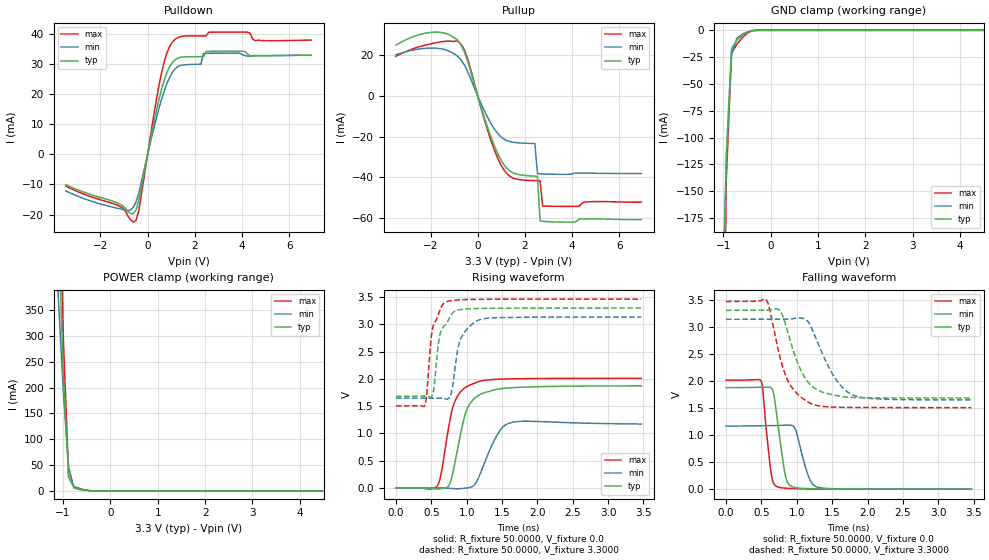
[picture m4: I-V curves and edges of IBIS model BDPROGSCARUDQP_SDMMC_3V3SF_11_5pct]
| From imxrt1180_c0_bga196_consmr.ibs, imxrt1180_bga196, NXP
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[Model]  BDPROGSCARUDQP_SDMMC_3V3SF_11_5pct
|   Model BDPROGSCARUDQP_SDMMC_3V3SF_11_5pct
| This model was characterised for following simulation conditions:
| External (pad) voltage:
|   - Typ: 3.3V,   - Min: 3.135V,   - Max: 3.465V
| Library cells for typ/min/max conditions are connected as defined below:
|  IO - External Pad
|  A - Core Input
|  EN - Output Buffer Enable
|  ASRCN3V3[0] - REFH3V3
|  ASRCN3V3[1] - REFH3V3 REFH3V3 gnde
|  ASRCN3V3[2] - gnde
|  ASRCN3V3[3] - gnde REFH3V3 gnde
|  ASRCP3V3[0] - vdde3v3 REFL3V3 REFL3V3
|  ASRCP3V3[1] - vdde3v3 REFL3V3 vdde3v3
|  ASRCP3V3[2] - REFL3V3 vdde3v3 vdde3v3
|  ASRCP3V3[3] - REFL3V3 REFL3V3 vdde3v3
|  IOGC - NC
|  PDN - vdd
|  PDRV - vdd
|  PSW - vdd
|  PUN - vdd
|  REFH3V3 - REFH3V3
|  REFL3V3 - REFL3V3
|  ZI - NC
|  gnd - gnd
|  gnde - gnde
|  vdd - vdd
|  vdde3v3 - vdde3v3
| All other pins connected to ground
Model_type I/O
Polarity   Non-Inverting
Enable   Active-Low
Vinl =   0.7500V
Vinh =   2.2500V
Vmeas =  1.6500V
Cref =   30.0000pF
Rref =   1.0000M
Vref =   3.3000V
C_comp   2.0930pF   2.0578pF   2.1401pF
|C_comp_pullup   0.3785pF   0.3910pF   0.3686pF
|C_comp_pulldown   0.6262pF   0.6569pF   0.6008pF
[Model Spec]
| variable   typ   min   max
Vinh   2.0625V   1.9594V   2.1656V
Vinl   0.8250V   0.7837V   0.8662V
[Temperature Range]   25.0000   0.1050k   -20.0000
[Voltage Range]   3.3000V   3.1350V   3.4650V
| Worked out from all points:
|   slope of the pulldown table from 0 to 0.495 V, typ, clamps not added: 26.6 ohm
|   slope of the pullup table from 0 to 0.495 V, typ, clamps not added: 27.4 ohm
|   GND clamp passes 1 mA (typ) near -0.44 V on its own axis
|   POWER clamp passes 1 mA (typ) near -0.50 V on its own axis
|   rising waveform, R_fixture 50.0000, V_fixture 0.0: 20-80 % time 205ps typ, 233ps min, 182ps max; typ from 0 V to 1.87 V
|   rising waveform, R_fixture 50.0000, V_fixture 3.3000: 20-80 % time 135ps typ, 150ps min, 118ps max; typ from 1.68 V to 3.3 V
|   falling waveform, R_fixture 50.0000, V_fixture 0.0: 20-80 % time 117ps typ, 148ps min, 91.5ps max; typ from 1.87 V to 0 V
|   falling waveform, R_fixture 50.0000, V_fixture 3.3000: 20-80 % time 287ps typ, 345ps min, 265ps max; typ from 3.3 V to 1.68 V
[Pulldown]
|Voltage   I(typ)   I(min)   I(max)
-3.465V   -10.11mA   -12.17mA   -10.6mA
-1.265V   -16.2mA    -17.95mA   -16.95mA
-825mV    -19.13mA   -18.72mA   -20.63mA
-495mV    -18.52mA   -15.93mA   -22.02mA
-385mV    -15.6mA    -13.21mA   -19.08mA
605mV     22.01mA    18.62mA    27.55mA
935mV     29.11mA    25.6mA     35.8mA
1.265V    31.87mA    29.03mA    38.66mA
2.255V    32.42mA    29.89mA    39.32mA
2.365V    32.42mA    33.45mA    39.32mA
4.235V    33.22mA    32.6mA     40.55mA
6.93V     32.91mA    32.89mA    37.89mA
[Pullup]
|Voltage   I(typ)   I(min)   I(max)
-3.465V   25.08mA    20.28mA    19.51mA
-1.87V    31.46mA    23.61mA    26.01mA
-770mV    26.31mA    18.66mA    26.34mA
-440mV    17.63mA    12.39mA    18.91mA
440mV     -16.26mA   -11.03mA   -17.69mA
990mV     -31.64mA   -20.2mA    -34.13mA
1.43V     -37.49mA   -22.68mA   -40.08mA
2.42V     -39.53mA   -23.48mA   -41.75mA
2.53V     -39.59mA   -38.31mA   -41.8mA
2.64V     -61.57mA   -38.4mA    -41.84mA
2.75V     -61.74mA   -38.47mA   -54.29mA
6.93V     -60.97mA   -38.21mA   -52.37mA
[GND_clamp]
|Voltage   I(typ)   I(min)   I(max)
-3.465V   -6.61A     -3.74A     -10.67A
-1.045V   -379.3mA   -292.6mA   -527.3mA
-935mV    -115.6mA   -121.5mA   -138.8mA
-825mV    -17.39mA   -23.01mA   -21.23mA
-715mV    -9.283mA   -7.4mA     -13.11mA
-605mV    -4.963mA   -3.854mA   -7.31mA
-495mV    -1.742mA   -1.524mA   -2.691mA
-385mV    -190.8uA   -276.7uA   -290.1uA
-275mV    -4.391uA   -16.17uA   -3.827uA
6.93V     0A         0A         0A
[POWER_clamp]
|Voltage   I(typ)   I(min)   I(max)
-3.465V   6.781A     3.823A     11A
-1.1V     518.6mA    375.5mA    743.7mA
-990mV    215.3mA    186.8mA    288.2mA
-880mV    27.02mA    45.34mA    26.73mA
-770mV    6.184mA    6.16mA     8.549mA
-550mV    1.523mA    1.344mA    2.266mA
-330mV    50.46uA    94.19uA    71.53uA
6.93V     0A         0A         0A
[Ramp]
| variable   typ   min   max
dV/dt_r  1.1232/0.2054n   0.7031/0.2325n   1.2067/0.1820n
dV/dt_f  0.9710/0.2867n   0.8923/0.3453n   1.1763/0.2645n
R_load = 50.0000
[Rising Waveform]
R_fixture= 50.0000
V_fixture= 0.0
V_fixture_min= 0.0
V_fixture_max= 0.0
|time   V(typ)   V(min)   V(max)
0s        34.73nV    367.6nV    81.7nV
578.6ps   -21.54mV   -41.18uV   26.19mV
636.9ps   -12.57mV   -1.034mV   243.5mV
741.3ps   32.17mV    -5.698mV   1.082V
848.5ps   561.5mV    -16.9mV    1.631V
964.1ps   1.279V     -6.169mV   1.826V
1.044ns   1.538V     6.864mV    1.886V
1.438ns   1.812V     987.2mV    1.994V
1.597ns   1.835V     1.185V     2.001V
3.47ns    1.872V     1.172V     2.011V
[Rising Waveform]
R_fixture= 50.0000
V_fixture= 3.3000
V_fixture_min= 3.1350
V_fixture_max= 3.4650
|time   V(typ)   V(min)   V(max)
0s        1.681V     1.647V     1.504V
405ps     1.684V     1.647V     1.509V
435ps     1.683V     1.647V     1.711V
518.9ps   1.718V     1.648V     2.927V
612.3ps   2.748V     1.648V     3.226V
705.1ps   3.001V     1.63V      3.411V
785.2ps   3.182V     1.756V     3.437V
918.1ps   3.273V     2.741V     3.452V
1.166ns   3.292V     3.078V     3.46V
3.47ns    3.3V       3.135V     3.465V
[Falling Waveform]
R_fixture= 50.0000
V_fixture= 0.0
V_fixture_min= 0.0
V_fixture_max= 0.0
|time   V(typ)   V(min)   V(max)
0s        1.873V     1.165V     2.011V
498.6ps   1.881V     1.171V     1.99V
634.5ps   1.873V     1.173V     319.4mV
673.1ps   1.761V     1.173V     108.7mV
720.8ps   1.319V     1.175V     46.33mV
840.4ps   242.4mV    1.181V     17.72mV
936.2ps   43.63mV    1.173V     11.23mV
1.174ns   9.797mV    209.9mV    5.009mV
1.283ns   6.926mV    41.77mV    3.634mV
3.47ns    119.1uV    230.3uV    66.52uV
[Falling Waveform]
R_fixture= 50.0000
V_fixture= 3.3000
V_fixture_min= 3.1350
V_fixture_max= 3.4650
|time   V(typ)   V(min)   V(max)
0s        3.3V       3.135V     3.465V
567.3ps   3.302V     3.135V     3.497V
614.5ps   3.305V     3.136V     3.329V
755.7ps   3.302V     3.137V     2.468V
862.5ps   2.941V     3.137V     2.034V
1.035ns   2.26V      3.162V     1.726V
1.197ns   1.92V      3.006V     1.582V
1.512ns   1.74V      2.111V     1.515V
1.784ns   1.694V     1.745V     1.508V
3.47ns    1.682V     1.648V     1.504V
